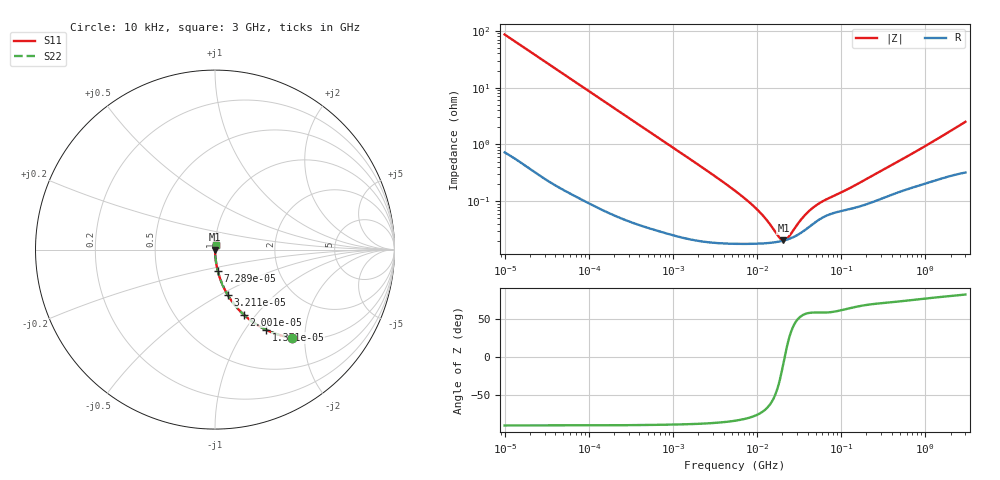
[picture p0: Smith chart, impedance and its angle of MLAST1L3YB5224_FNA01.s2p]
! MLAST1L3YB5224_FNA01  S-PARAMETER MODEL  ( Standard Model )
! Model Generated by TAIYO YUDEN Corporation (http://www.ty-top.com)
! Version 1.0
! TAIYO YUDEN Control No. 220601
! Copyright(c) 2010 TAIYO YUDEN CO.,LTD. All Rights Reserved.
! Product Description (link to TY-COMPAS)
! https://ds.yuden.co.jp/TYCOMPAS/or/detail?pn=MLAST1L3YB5224KFNA01&u=M
! Products Name : Multilayer Ceramic Capacitors
! Characteristics :
!  Capacitance : 0.22 [uF] , Rated Voltage : 25 [V] , TCC : X5R
!  Case Size : 1.0 x 0.5 / 0.039 x 0.02 [mm/inch] , Thickness : 0.3 / 0.012 [mm/inch]
!  (Conditions: Temperature = 25 [degC] , DC Bias Voltage = 0 [V])
! External Node Assignments :
!  1  o---| |---o  2
! GND o---------o GND
! Frequency Range : 10kHz  -  3GHz  [ 401 STEP ]
# MHZ S RI R 50
! Freq[MHz].  S11 Real  S11 Imag  S21 Real  S21 Imag  S12 Real  S12 Imag  S22 Real  S22 Imag
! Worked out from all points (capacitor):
!   401 points, 10 kHz to 3 GHz, reference 50 ohm
!   read as one part in series: C = 184 nF near 10.65 kHz
!   lowest |Z| = 20.5 mohm at 20.59 MHz (marker M1)
!   series resonance near 21.3 MHz, so ESL is about 300 pH
!   S11 on the Smith chart (normalised r, x): 10 kHz: 1.01, -1.72; 13.71 kHz: 1.01, -1.26; 20.01 kHz: 1.01, -0.87; 32.11 kHz: 1.00, -0.54; 72.89 kHz: 1.00, -0.24; 3 GHz: 1.01, +0.05
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0.01  0.4272 -0.4905  0.5728 0.4905  0.5728 0.4905  0.4272 -0.4905
0.013707  0.2862 -0.4477  0.7138 0.4477  0.7138 0.4477  0.2862 -0.4477
0.02001  0.16 -0.3623  0.84 0.3623  0.84 0.3623  0.16 -0.3623
0.03211  0.07 -0.2509  0.93 0.2509  0.93 0.2509  0.07 -0.2509
0.072886  0.0152 -0.1176  0.9848 0.1176  0.9848 0.1176  0.0152 -0.1176
0.082683  0.012 -0.1041  0.988 0.1041  0.988 0.1041  0.012 -0.1041
0.199902  0.00248 -0.0437  0.9975 0.0437  0.9975 0.0437  0.00248 -0.0437
0.683653  0.000464 -0.0129  0.9995 0.0129  0.9995 0.0129  0.000464 -0.0129
2.570001  0.000203 -0.00342  0.9998 0.00342  0.9998 0.00342  0.000203 -0.00342
5.477226  0.000181 -0.00152  0.9998 0.00152  0.9998 0.00152  0.000181 -0.00152
10.29003  0.00018 -0.000668  0.9998 0.000668  0.9998 0.000668  0.00018 -0.000668
13.24217  0.000184 -0.000416  0.9998 0.000416  0.9998 0.000416  0.000184 -0.000416
18.15044  0.000195 -0.000136  0.9998 0.000136  0.9998 0.000136  0.000195 -0.000136
20.5901  0.000203 -2.89e-05  0.9998 2.89e-05  0.9998 2.89e-05  0.000203 -2.89e-05
21.93027  0.000208 2.46e-05  0.9998 -2.46e-05  0.9998 -2.46e-05  0.000208 2.46e-05
23.35767  0.000215 7.8e-05  0.9998 -7.8e-05  0.9998 -7.8e-05  0.000215 7.8e-05
34.09912  0.000285 0.000405  0.9997 -0.000405  0.9997 -0.000405  0.000285 0.000405
45.28751  0.000389 0.000644  0.9996 -0.000644  0.9996 -0.000644  0.000389 0.000644
60.14696  0.000516 0.000854  0.9995 -0.000854  0.9995 -0.000854  0.000516 0.000854
132.292  0.000743 0.0016  0.9993 -0.0016  0.9993 -0.0016  0.000743 0.0016
374.4521  0.00127 0.00393  0.9987 -0.00393  0.9987 -0.00393  0.00127 0.00393
3000  0.00381 0.0247  0.9962 -0.0247  0.9962 -0.0247  0.00381 0.0247
